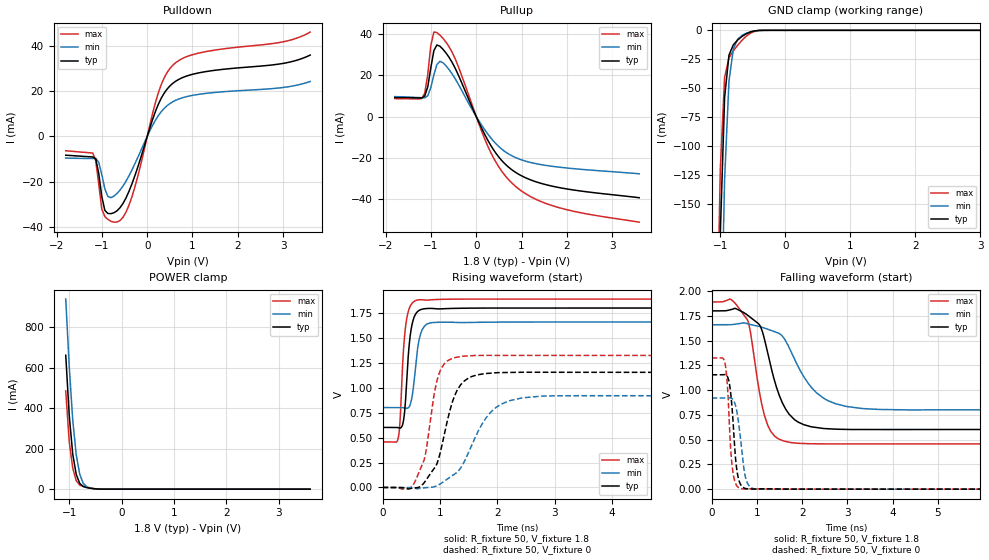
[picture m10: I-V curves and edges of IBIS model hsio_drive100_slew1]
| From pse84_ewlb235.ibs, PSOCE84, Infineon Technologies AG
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[Model] hsio_drive100_slew1
Model_type I/O
Enable   Active-High
Vinl  =  0.54
Vinh  =  1.26
Vmeas =  0.9
Cref  =  15pF
| Capacitance   typ   min   max
C_comp   1.183861e-12   1.145095e-12   1.230403e-12
| Variables   typ   min   max
[GND Clamp Reference]   0   0   0
[POWER Clamp Reference]   1.8   1.66   1.89
[Pulldown Reference]   0   0   0
[Pullup Reference]   1.8   1.66   1.89
[Temperature Range]   25   125   -40
[Voltage Range]   1.8   1.66   1.89
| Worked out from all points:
|   slope of the pulldown table from 0 to 0.27 V, typ, clamps not added: 17.8 ohm
|   slope of the pullup table from 0 to 0.27 V, typ, clamps not added: 22.5 ohm
|   GND clamp passes 1 mA (typ) near -0.51 V on its own axis
|   POWER clamp passes 1 mA (typ) near -0.47 V on its own axis
|   falling waveform, R_fixture 50, V_fixture 1.8: 20-80 % time 455ps typ, 672ps min, 317ps max; typ from 1.8 V to 0.602 V
|   falling waveform, R_fixture 50, V_fixture 0: 20-80 % time 115ps typ, 146ps min, 98.5ps max; typ from 1.16 V to 0 V
|   rising waveform, R_fixture 50, V_fixture 1.8: 20-80 % time 94.2ps typ, 109ps min, 86.2ps max; typ from 0.602 V to 1.8 V
|   rising waveform, R_fixture 50, V_fixture 0: 20-80 % time 317ps typ, 510ps min, 225ps max; typ from 0 V to 1.16 V
[GND Clamp]
| Voltage   I(typ)   I(min)   I(max)
-1.137V   -688mA     -831.1mA   -596.4mA
-1.07V    -398.5mA   -545.5mA   -312.5mA
-1.003V   -176.8mA   -300mA     -120.9mA
-936.6mV  -57.93mA   -128.6mA   -40.51mA
-869.7mV  -21.44mA   -44.12mA   -23.78mA
-802.8mV  -12.54mA   -16.03mA   -17.79mA
-735.9mV  -8.37mA    -7.69mA    -12.93mA
-669mV    -5.28mA    -4.356mA   -8.606mA
-535.2mV  -1.316mA   -1.208mA   -2.332mA
-401.4mV  -73.56uA   -132.2uA   -119.3uA
3.6V      0A         0A         0A
[POWER Clamp]
| Voltage   I(typ)   I(min)   I(max)
-1.07V    662.2mA    940mA      485.7mA
-1.003V   363.7mA    605.6mA    233mA
-936.6mV  172.7mA    341mA      103.9mA
-869.7mV  72.74mA    168.6mA    41.65mA
-802.8mV  28.31mA    73.56mA    19.99mA
-735.9mV  13.11mA    28.55mA    13.36mA
-669mV    7.76mA     11.5mA     8.963mA
-535.2mV  2.357mA    2.863mA    2.668mA
-334.5mV  34.33uA    127.4uA    15.59uA
3.6V      0A         0A         0A
[Pulldown]
| Voltage   I(typ)   I(min)   I(max)
-1.8V     -8.273mA   -9.546mA   -6.313mA
-1.204V   -9.042mA   -9.718mA   -7.313mA
-1.137V   -9.896mA   -9.717mA   -10.71mA
-1.003V   -26.52mA   -16.83mA   -32.08mA
-936.6mV  -32.58mA   -23.08mA   -35.3mA
-869.7mV  -33.95mA   -26.47mA   -36.57mA
-669mV    -32.79mA   -25.19mA   -37.75mA
-401.4mV  -24.12mA   -17.29mA   -30.21mA
248.3mV   14.29mA    9.245mA    19.39mA
558.6mV   23.29mA    15.2mA     31.23mA
1.117V    27.91mA    18.49mA    36.62mA
3.6V      35.84mA    24.21mA    45.97mA
[Pullup]
| Voltage   I(typ)   I(min)   I(max)
-1.8V     9.249mA    9.655mA    8.684mA
-1.204V   8.988mA    9.128mA    8.718mA
-1.137V   9.935mA    9.053mA    11.31mA
-1.07V    14.47mA    10.11mA    20.5mA
-1.003V   23.56mA    14.04mA    34.37mA
-936.6mV  31.85mA    20.11mA    40.84mA
-869.7mV  34.6mA     25.14mA    40.62mA
-468.3mV  23.5mA     18.41mA    28.09mA
310.3mV   -13.54mA   -10.01mA   -16.89mA
806.9mV   -26.03mA   -19.17mA   -32.53mA
1.738V    -33.91mA   -24.2mA    -43.44mA
3.6V      -39.23mA   -27.66mA   -51.05mA
[Ramp]
dV/dt_r   0.692748/0.316942n  0.551907/0.51009n  0.794721/0.225422n
dV/dt_f   0.718532/0.455453n  0.515083/0.672415n  0.859883/0.316509n
R_load = 50
[Falling Waveform]
R_fixture = 50
V_fixture = 1.8
V_fixture_min = 1.66
V_fixture_max = 1.89
| Time   V(typ)   V(min)   V(max)
0s        1.8V       1.66V      1.89V
420.1ps   1.812V     1.661V     1.917V
793.1ps   1.758V     1.67V      1.708V
1.058ns   1.659V     1.643V     979mV
1.306ns   1.248V     1.604V     585.4mV
1.551ns   883.8mV    1.551V     493.7mV
1.91ns    678mV      1.242V     463.2mV
2.58ns    609.5mV    892.2mV    456.8mV
3.714ns   601.9mV    804.7mV    456.9mV
50ns      602.4mV    801.5mV    456.9mV
[Falling Waveform]
R_fixture = 50
V_fixture = 0
V_fixture_min = 0
V_fixture_max = 0
| Time   V(typ)   V(min)   V(max)
0s        1.155V     919.8mV    1.325V
282.2ps   1.157V     919.8mV    1.296V
374.8ps   1.107V     922.3mV    849.6mV
428ps     946.7mV    920.6mV    364.9mV
482.6ps   631.1mV    898.6mV    140.2mV
565.1ps   172.4mV    767.7mV    29.51mV
695.1ps   18.32mV    276.6mV    2.401mV
806.5ps   2.745mV    47.31mV    3.105mV
1.027ns   2.045mV    777.2uV    1.576mV
50ns      14.72nV    1.039uV    5.426nV
[Rising Waveform]
R_fixture = 50
V_fixture = 1.8
V_fixture_min = 1.66
V_fixture_max = 1.89
| Time   V(typ)   V(min)   V(max)
0s        602.4mV    801.5mV    456.9mV
271.7ps   600.2mV    801.5mV    489.9mV
306.4ps   596.7mV    801.6mV    677.6mV
348.7ps   628.2mV    801mV      1.214V
410.5ps   959.6mV    794.3mV    1.655V
450.3ps   1.334V     799.7mV    1.768V
494.1ps   1.572V     854mV      1.831V
657ps     1.782V     1.528V     1.884V
1.093ns   1.794V     1.658V     1.888V
50ns      1.8V       1.66V      1.89V
[Rising Waveform]
R_fixture = 50
V_fixture = 0
V_fixture_min = 0
V_fixture_max = 0
| Time   V(typ)   V(min)   V(max)
0s        14.74nV    1.033uV    5.346nV
491.1ps   -9.212mV   -2.991mV   378.5uV
718.4ps   42.21mV    -3.332mV   264.1mV
901.1ps   189.6mV    6.726mV    938.7mV
1.028ns   402.6mV    42.91mV    1.198V
1.259ns   922.8mV    134.1mV    1.303V
1.582ns   1.118V     458.7mV    1.324V
2.063ns   1.152V     833.6mV    1.325V
3ns       1.155V     919.6mV    1.324V
50ns      1.155V     919.8mV    1.325V
